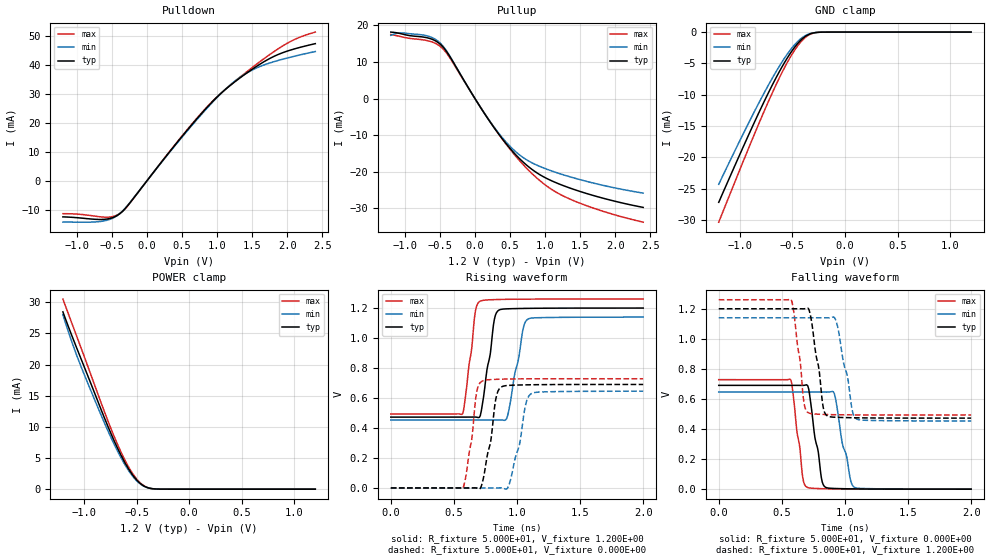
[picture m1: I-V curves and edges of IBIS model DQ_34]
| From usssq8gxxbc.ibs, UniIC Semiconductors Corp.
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|   Model DQ_34
[Model] DQ_34
Model_type I/O
Polarity   Non-Inverting
Enable   Active-High
Vinl =  8.300E-01
Vinh =  9.700E-01
Vmeas =  8.400E-01
Rref =  5.000E+01
Vref =  1.200E+00
C_comp   6.304E-13   6.246E-13   6.399E-13
C_comp_pullup   3.076E-13   3.061E-13   3.099E-13
C_comp_pulldown   3.075E-13   2.994E-13   3.185E-13
[Model Spec]
Vinh   9.700E-01   9.250E-01   1.015E+00
Vinl   8.300E-01   7.850E-01   8.750E-01
Vmeas   8.400E-01   7.980E-01   8.820E-01
Vref   1.200E+00   1.140E+00   1.260E+00
Rref   5.000E+01   5.000E+01   5.000E+01
[Temperature Range]   4.500E+01   9.500E+01   0.000E+00
[Voltage Range]   1.200E+00   1.140E+00   1.260E+00
[C Comp Corner]
C_comp_pullup   3.076E-13   3.099E-13   3.061E-13
C_comp_pulldown   3.075E-13   2.994E-13   3.185E-13
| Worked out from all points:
|   slope of the pulldown table from 0 to 0.18 V, typ, clamps not added: 31.9 ohm
|   slope of the pullup table from 0 to 0.18 V, typ, clamps not added: 33.5 ohm
|   GND clamp passes 1 mA (typ) near -0.40 V on its own axis
|   POWER clamp passes 1 mA (typ) near -0.47 V on its own axis
|   rising waveform, R_fixture 5.000E+01, V_fixture 1.200E+00: 20-80 % time 72.1ps typ, 85.7ps min, 62.3ps max; typ from 0.473 V to 1.2 V
|   rising waveform, R_fixture 5.000E+01, V_fixture 0.000E+00: 20-80 % time 75.4ps typ, 91.2ps min, 64ps max; typ from 0 V to 0.691 V
|   falling waveform, R_fixture 5.000E+01, V_fixture 0.000E+00: 20-80 % time 71.4ps typ, 87.7ps min, 60.4ps max; typ from 0.691 V to 0 V
|   falling waveform, R_fixture 5.000E+01, V_fixture 1.200E+00: 20-80 % time 70.2ps typ, 86.1ps min, 60.1ps max; typ from 1.2 V to 0.473 V
[Pulldown]
|Voltage   I(typ)   I(min)   I(max)
-1.2V     -12.53mA   -14.32mA   -11.42mA
-645mV    -13.42mA   -14.06mA   -12.56mA
-497mV    -12.85mA   -13.06mA   -12.46mA
-386mV    -11.39mA   -11.34mA   -11.31mA
-275mV    -8.623mA   -8.476mA   -8.696mA
687mV     20.77mA    20.48mA    20.97mA
983mV     28.6mA     28.43mA    28.7mA
1.205V    33.35mA    33.56mA    33.46mA
1.464V    38mA       37.89mA    38.52mA
1.797V    42.91mA    41.13mA    44.49mA
2.093V    45.59mA    43.06mA    48.79mA
2.4V      47.47mA    44.75mA    51.48mA
[Pullup]
|Voltage   I(typ)   I(min)   I(max)
-1.2V     18.14mA    17.25mA    17.49mA
-1.041V   17.62mA    17.9mA     16.82mA
-745mV    16.8mA     17.35mA    16.03mA
-486mV    14.66mA    14.96mA    14.08mA
-375mV    11.98mA    12.11mA    11.6mA
32mV      -984.3uA   -981.2uA   -967.7uA
291mV     -8.438mA   -8.271mA   -8.42mA
513mV     -13.89mA   -13.28mA   -14.13mA
735mV     -18.15mA   -16.71mA   -18.99mA
1.031V    -21.89mA   -19.33mA   -23.98mA
1.327V    -24.24mA   -21.21mA   -27.2mA
2.4V      -29.72mA   -25.82mA   -33.75mA
[GND_clamp]
|Voltage   I(typ)   I(min)   I(max)
-1.2V     -27.2mA    -24.33mA   -30.38mA
-875mV    -14.93mA   -13.17mA   -16.89mA
-750mV    -10.47mA   -9.157mA   -11.95mA
-650mV    -7.145mA   -6.184mA   -8.244mA
-575mV    -4.884mA   -4.175mA   -5.699mA
-500mV    -2.92mA    -2.45mA    -3.459mA
-425mV    -1.383mA   -1.13mA    -1.679mA
-375mV    -673.2uA   -542.8uA   -837uA
-300mV    -135.5uA   -116.3uA   -166.1uA
-225mV    -14.67uA   -15.93uA   -14.24uA
1.2V      0A         0A         0A
[POWER_clamp]
|Voltage   I(typ)   I(min)   I(max)
-1.2V     28.45mA    28mA       30.5mA
-1.125V   25.07mA    24.12mA    27.08mA
-1.025V   20.8mA     19.57mA    22.55mA
-850mV    13.34mA    12.42mA    14.46mA
-750mV    9.2mA      8.545mA    10.01mA
-650mV    5.523mA    5.115mA    6.037mA
-575mV    3.235mA    2.981mA    3.547mA
-500mV    1.501mA    1.371mA    1.657mA
-450mV    723.1uA    662.7uA    804.4uA
-375mV    148.3uA    148.7uA    156.1uA
-300mV    17.6uA     22.56uA    14.19uA
1.2V      0A         0A         0A
[Ramp]
| variable   typ   min   max
dV/dt_r   4.143E-01/7.585E-11   3.874E-01/9.177E-11   4.371E-01/6.407E-11
dV/dt_f   4.364E-01/7.029E-11   4.120E-01/8.641E-11   4.599E-01/6.040E-11
R_load = 5.000E+01
[Rising Waveform]
R_fixture= 5.000E+01
V_fixture= 1.200E+00
V_fixture_min= 1.140E+00
V_fixture_max= 1.260E+00
|time   V(typ)   V(min)   V(max)
0s        472.6mV    453.2mV    493.5mV
566ps     472.7mV    453.2mV    491.9mV
669ps     473.1mV    453.3mV    1.172V
709ps     482.7mV    453.3mV    1.246V
820ps     1.122V     453.4mV    1.256V
857ps     1.187V     453.6mV    1.257V
925ps     1.195V     480.1mV    1.258V
1.046ns   1.197V     1.052V     1.259V
1.079ns   1.198V     1.122V     1.259V
2ns       1.2V       1.14V      1.26V
[Rising Waveform]
R_fixture= 5.000E+01
V_fixture= 0.000E+00
V_fixture_min= 0.000E+00
V_fixture_max= 0.000E+00
|time   V(typ)   V(min)   V(max)
0s        192.9nV    543.7nV    98.81nV
571ps     85.53uV    27.09uV    -2.027mV
643ps     250.1uV    51.12uV    335mV
680ps     -660.3uV   74.9uV     637.9mV
727ps     41.26mV    67.73uV    713.6mV
831ps     589.6mV    156uV      724.4mV
874ps     672.5mV    564.7uV    725.6mV
943ps     684.5mV    37.72mV    726.8mV
1.106ns   688.3mV    624.6mV    728.1mV
2ns       690.5mV    645.7mV    728.5mV
[Falling Waveform]
R_fixture= 5.000E+01
V_fixture= 0.000E+00
V_fixture_min= 0.000E+00
V_fixture_max= 0.000E+00
|time   V(typ)   V(min)   V(max)
0s        690.5mV    645.8mV    728.5mV
566ps     690.5mV    645.8mV    731.5mV
666ps     690.3mV    645.8mV    77.03mV
699ps     692.6mV    645.8mV    13.04mV
813ps     77.11mV    645.8mV    3.331mV
847ps     12.14mV    645.6mV    2.522mV
917ps     4.672mV    633.3mV    1.434mV
978ps     3.226mV    309.1mV    883.4uV
1.075ns   1.836mV    12.29mV    414.6uV
2ns       13.19uV    120.2uV    1.179uV
[Falling Waveform]
R_fixture= 5.000E+01
V_fixture= 1.200E+00
V_fixture_min= 1.140E+00
V_fixture_max= 1.260E+00
|time   V(typ)   V(min)   V(max)
0s        1.2V       1.14V      1.26V
573ps     1.2V       1.14V      1.262V
647ps     1.2V       1.14V      840.1mV
675ps     1.2V       1.14V      576.2mV
710ps     1.201V     1.14V      508.5mV
828ps     543.8mV    1.14V      497.3mV
854ps     491.5mV    1.14V      496.6mV
932ps     478mV      1.114V     495.1mV
1.085ns   474.8mV    471.3mV    494mV
2ns       472.6mV    453.4mV    493.5mV
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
